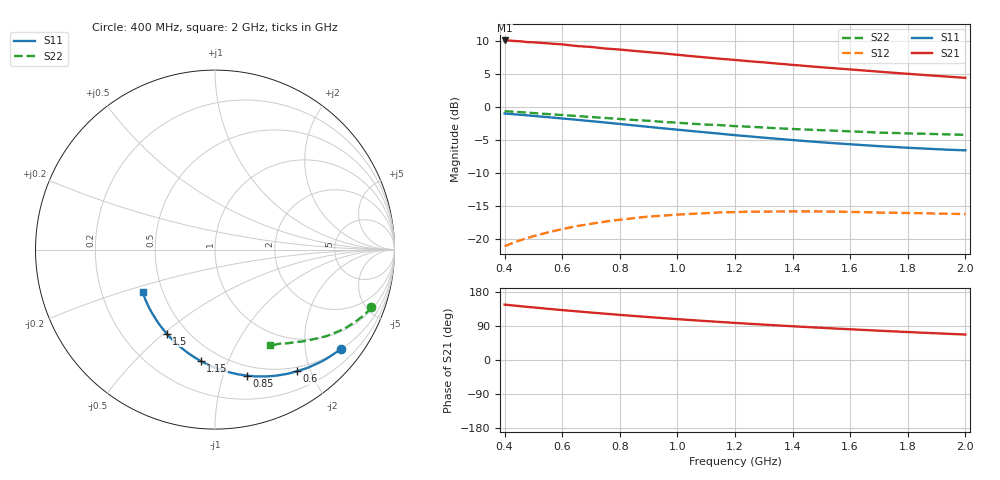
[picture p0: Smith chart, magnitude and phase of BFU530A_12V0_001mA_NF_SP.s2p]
! Filename:  P:\Prog\Test\Noise\ATS_data\Testdata_Net\06 Compressed Noise after Statistics\BFU530A_APG2013_33_A05_12p0V_001mA_SP_CM01_D.sf
! Date/Time: Tue 16/Apr/2013 15:10:54
! BFU530A_APG2013_33_A05_12p0V_1to25mA_NF_CM01_Bias1_R.sf
! Noise Parameter Data File
! BFU530A_APG2013_33_A05_12p0V_1to25mA_NF_CM01
! Date/time: Fri Apr 12 17:55:00 2013
! freq range =  0.4000 to  2.0000 GHz, 37 points
! bias range =  0.9950 to 24.9950 mA, 8 points
! bias supplies used: 1 1 0 0 0 0
! VAR bias_mode= 1  ! Specify V_out, I_out
! VAR bias_var = 1  ! Bias variable = I_out
! VAR V_out= 12.001000
! VAR I_out= 0.995000
! VAR V_in= 0.779100
! VAR I_in= 0.007599
! Device data file deembeded for feedlines and parallel
! Original file: \06 Compressed Noise after Statistics\BFU530A_APG2013_33_A05_12p0V_001mA_SP_CM01_R.sf
! Feed-files: PR017V01_150413_Feed1.s2p, PR017V01_150413_Feed2.s2p
! Parallel-file: PR017V01_150413_Par.s2p
# MHz S MA R 50
!  Freq-MHz  S11-mag  S11-arg  S21-mag  S21-arg  S12-mag  S12-arg  S22-mag  S22-arg
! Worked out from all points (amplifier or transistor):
!   37 points, 400 MHz to 2 GHz, reference 50 ohm
!   highest |S21| = 10.1 dB at 400 MHz (marker M1)
!   |S21| within 3 dB of that: start of sweep to 1.21 GHz
!   unconditionally stable (mu >= 1): nowhere
!   at 500 MHz: K = 0.23, MSG = 14.7 dB, |S12| = -19.6 dB
!   at 1.1 GHz: K = 0.47, MSG = 11.8 dB, |S12| = -16.1 dB
!   at 2 GHz: K = 0.88, MSG = 10.3 dB, |S12| = -16.3 dB
!   lowest NFmin = 0.55 dB at 420 MHz
!   S11 on the Smith chart (normalised r, x): 400 MHz: 0.51, -2.80; 600 MHz: 0.44, -1.80; 850 MHz: 0.41, -1.20; 1.15 GHz: 0.39, -0.80; 1.5 GHz: 0.39, -0.51; 2 GHz: 0.38, -0.24
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400  0.8926 -38.3  3.205 146.2  0.08773 65.6  0.9293 -20.3
440  0.8785 -42.0  3.172 143.1  0.09476 63.6  0.9185 -22.0
460  0.8714 -43.8  3.15 141.7  0.09811 62.5  0.9134 -22.9
480  0.8649 -45.4  3.114 140.2  0.1013 61.5  0.9065 -23.7
500  0.8567 -47.3  3.104 138.7  0.1044 60.6  0.9005 -24.5
550  0.8378 -51.7  3.047 135.2  0.1116 58.2  0.8843 -26.5
600  0.8185 -55.9  2.993 131.7  0.1182 56.0  0.8692 -28.4
650  0.8007 -59.9  2.907 128.5  0.1245 54.0  0.8555 -30.1
700  0.7811 -64.0  2.862 125.2  0.1298 51.9  0.8399 -31.9
750  0.763 -67.9  2.782 122.1  0.1349 50.1  0.8258 -33.4
800  0.7439 -71.9  2.733 119.1  0.1393 48.4  0.8115 -34.9
850  0.7247 -75.7  2.67 116.1  0.1433 46.7  0.7978 -36.4
950  0.6893 -83.2  2.557 110.5  0.1497 43.6  0.7714 -39.2
1050  0.657 -90.2  2.435 105.2  0.1544 41.1  0.7471 -41.7
1150  0.6266 -97.2  2.326 100.3  0.1585 38.8  0.7283 -43.9
1200  0.6118 -100.6  2.279 97.9  0.1591 37.9  0.7166 -45.1
1350  0.5733 -110.4  2.136 91.2  0.1609 35.6  0.6892 -48.3
1500  0.5401 -119.9  2.005 84.9  0.1609 34.0  0.6673 -51.2
1650  0.5127 -129.0  1.894 79.2  0.1591 33.4  0.6472 -54.1
1750  0.4976 -135.0  1.821 75.6  0.1575 33.6  0.6357 -55.7
1850  0.4846 -140.8  1.756 72.1  0.1561 34.0  0.6278 -57.5
2000  0.469 -149.4  1.666 67.2  0.1538 35.7  0.6149 -60.2
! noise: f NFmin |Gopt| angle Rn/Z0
400  0.5597  0.6315  20.9  0.3701
460  0.6186  0.6356  26.21  0.3685
600  0.6187  0.6229  32.8  0.3457
800  0.6612  0.5977  49.35  0.2709
1000  0.7074  0.5927  62.35  0.2451
1200  0.804  0.5969  73.06  0.2434
1400  0.8708  0.5707  88.27  0.1875
1600  0.8934  0.5476  102.1  0.15
1800  0.8318  0.5332  115.9  0.1044
2000  0.8233  0.5218  126.7  0.1054
